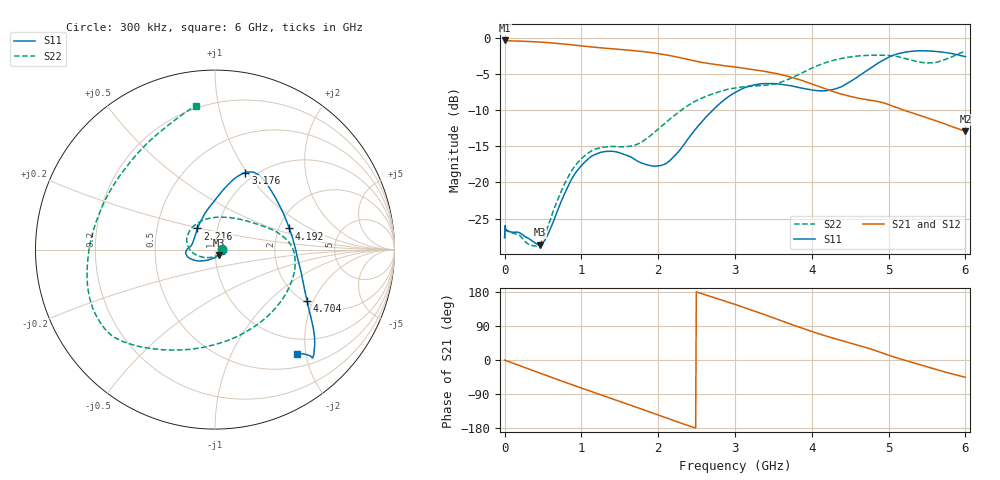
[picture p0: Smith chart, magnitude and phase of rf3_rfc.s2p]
!Agilent Technologies,M9375A,MY55441453,A.02.50.04
!Agilent M9375A: A.02.50.04
!Date: Monday, December 12, 2016 11:35:14
!Correction: S11(Full 2 Port(1,2))
!S21(Full 2 Port(1,2))
!S12(Full 2 Port(1,2))
!S22(Full 2 Port(1,2))
!S2P File: Measurements: S11, S21, S12, S22:
# Hz S  dB  R 50
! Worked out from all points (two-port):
!   751 points, 300 kHz to 6 GHz, reference 50 ohm
!   highest |S21| = -0.38 dB at 8.3 MHz (marker M1); lowest = -12.9 dB at 6 GHz (marker M2)
!   |S21| within 3 dB of the highest: start of sweep to 2.55 GHz
!   lowest |S11| = -28.6 dB at 456.3 MHz (marker M3), VSWR 1.08, Z = 52 - j3.22 ohm
!   |S11| at or under -10 dB: start of sweep to 2.711 GHz
!   |S22| runs from -28.8 to -1.8 dB; largest |S21 - S12| = 0.0041
!   S11 on the Smith chart (normalised r, x): 300 kHz: 1.09, -0.00; 2.216 GHz: 0.80, +0.19; 3.176 GHz: 0.90, +0.98; 4.192 GHz: 2.28, +0.66; 4.704 GHz: 2.06, -1.79; 6 GHz: 0.72, -1.84
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300000  -27.63 -2.4  -0.39 -0.1  -0.39 -0.1  -27.71 0.9
8299600  -25.95 3.3  -0.38 -0.6  -0.37 -0.4  -25.98 2.7
4.562772e8  -28.60 -56.3  -0.60 -34.3  -0.60 -34.3  -28.58 -85.7
5.522724e8  -27.43 -85.7  -0.66 -41.5  -0.66 -41.5  -26.44 -115.4
7.842608e8  -21.50 -133.3  -0.88 -58.5  -0.88 -58.6  -20.11 -159.3
1.00025e9  -17.66 -153.4  -1.13 -74.0  -1.13 -74.0  -16.71 176.3
1.224239e9  -15.93 -166.6  -1.37 -89.7  -1.37 -89.7  -15.26 152.4
1.488226e9  -15.87 -177.6  -1.60 -108.1  -1.60 -108.2  -15.07 118.4
2.0002e9  -17.71 156.6  -2.19 -145.3  -2.19 -145.4  -12.62 43.7
2.216189e9  -16.29 129.7  -2.61 -161.0  -2.60 -161.0  -10.69 27.3
2.59217e9  -11.31 90.7  -3.46 173.7  -3.45 173.6  -8.23 10.7
3.00015e9  -7.57 73.8  -4.04 146.8  -4.04 146.7  -6.94 -7.2
3.176141e9  -6.72 68.5  -4.30 134.5  -4.30 134.4  -6.71 -20.9
3.40013e9  -6.33 62.4  -4.68 118.5  -4.67 118.4  -6.56 -45.8
3.640118e9  -6.50 55.0  -5.20 100.9  -5.20 100.8  -5.98 -77.4
4.0001e9  -7.22 34.4  -6.37 75.2  -6.37 75.1  -4.20 -114.9
4.19209e9  -7.32 15.9  -7.11 62.9  -7.11 62.8  -3.40 -126.4
4.704065e9  -4.63 -29.0  -8.53 33.1  -8.53 33.0  -2.45 -142.9
5.00005e9  -2.69 -41.0  -9.23 12.7  -9.23 12.6  -2.45 -154.7
5.40803e9  -1.80 -47.8  -10.74 -12.5  -10.73 -12.7  -3.37 165.1
5.720014e9  -2.03 -48.3  -11.86 -31.0  -11.85 -31.1  -3.07 122.7
6e9  -2.62 -51.7  -12.91 -45.5  -12.91 -45.7  -1.84 97.7
